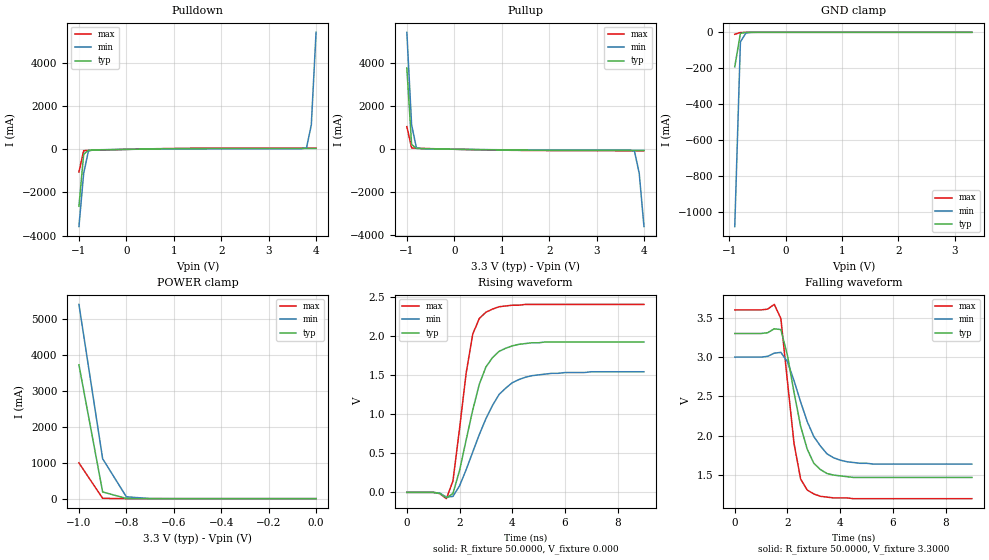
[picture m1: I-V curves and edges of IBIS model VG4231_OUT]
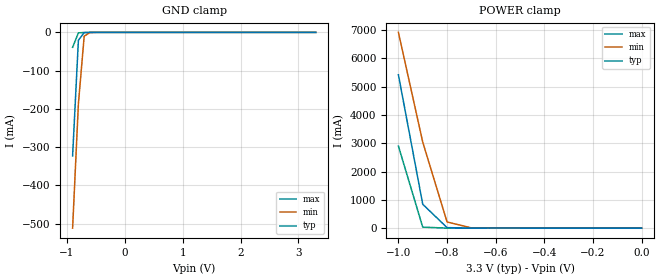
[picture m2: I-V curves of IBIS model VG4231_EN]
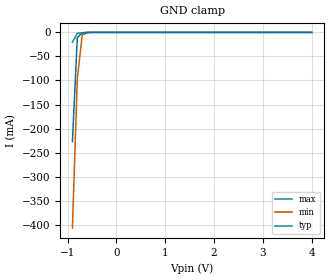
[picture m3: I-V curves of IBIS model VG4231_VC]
[IBIS ver]   2.1
[File name]   423bcacm.ibs
[File Rev]   0.1
[Date]   November 12, 2007
[Copyright]   EPSONTOYOCOM Corp.
|   Component VG-4231CAxxC
[Component]   VG-4231CAxxC
[Manufacturer]   EPSONTOYOCOM Corp.
[Package]
| variable   typ   min   max
R_pkg   0.20   0.13   0.28
L_pkg   5.16nH   4.56nH   5.76nH
C_pkg   1.23pF   1.03pF   1.53pF
[Pin]  signal_name   model_name   R_pin   L_pin   C_pin
1   VC   VG4231_VC
2   NC   NC
3   GND   GND
4   OUT   VG4231_OUT
5   OE   VG4231_EN
6   VDD   POWER
| Models and submodels in the file (3): VG4231_OUT (3-state), VG4231_EN (Input), VG4231_VC (Input)
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|   Model VG4231_OUT
[Model]   VG4231_OUT
Model_type   3-state
Polarity   Non-Inverting
Enable   Active-High
C_comp   2.2010pF   2.2010pF   2.2010pF
[Temperature Range]   27.0000   85.0000   -40.0000
[Voltage Range]   3.3000V   3.0000V   3.6000V
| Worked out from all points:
|   slope of the pulldown table from 0 to 0.495 V, typ, clamps not added: 28.4 ohm
|   slope of the pullup table from 0 to 0.495 V, typ, clamps not added: 27.7 ohm
|   GND clamp passes 1 mA (typ) near -0.71 V on its own axis
|   POWER clamp passes 1 mA (typ) near -0.71 V on its own axis
|   rising waveform, R_fixture 50.0000, V_fixture 0.000: 20-80 % time 860ps typ, 1.2ns min, 575ps max; typ from 0 V to 1.92 V
|   falling waveform, R_fixture 50.0000, V_fixture 3.3000: 20-80 % time 699ps typ, 942ps min, 507ps max; typ from 3.3 V to 1.47 V
[Pulldown]
| voltage   I(typ)   I(min)   I(max)
-1V       -2.64A     -3.58A     -1.05A
-900mV    -227mA     -1.11A     -59.8mA
-800mV    -37.8mA    -77.2mA    -45.4mA
-600mV    -24.7mA    -18.8mA    -34.3mA
1.2V      33.1mA     23.8mA     47.8mA
3.6V      41.7mA     29.9mA     59.7mA
3.8V      41.8mA     81.9mA     59.8mA
3.9V      41.9mA     1.14A      59.9mA
4V        42.4mA     5.43A      59.9mA
[Pullup]
| voltage   I(typ)   I(min)   I(max)
-1V       3.77A      5.43A      1.05A
-900mV    225mA      1.14A      61.1mA
-800mV    40.2mA     79.9mA     46.3mA
-700mV    30.8mA     27.5mA     40.2mA
-500mV    21.5mA     17.4mA     28.5mA
1.3V      -37.2mA    -28.9mA    -50.6mA
3.6V      -50.6mA    -38.5mA    -69.6mA
3.8V      -50.9mA    -91.7mA    -69.9mA
3.9V      -51.2mA    -1.12A     -70.1mA
4V        -51.8mA    -3.59A     -70.3mA
[GND_clamp]
| voltage   I(typ)   I(min)   I(max)
-900mV    -192mA     -1.08A     -11mA
-800mV    -5.99mA    -53.3mA    -1.09mA
-700mV    -646uA     -3.06mA    -314uA
3.3V      11.8pA     1.53uA     9pA
[POWER_clamp]
| voltage   I(typ)   I(min)   I(max)
-1V       3.72A      5.4A       997mA
-900mV    187mA      1.11A      9.61mA
-800mV    5.59mA     52.3mA     343uA
-700mV    457uA      3.17mA     42.4uA
-600mV    78.5uA     431uA      4.29uA
-500mV    10.7uA     85.5uA     259nA
-400mV    1.01uA     13.3uA     7.61nA
-300mV    59.2nA     1.53uA     157pA
-200mV    2.41nA     123nA      14.1pA
-100mV    84.8pA     7.1nA      11.4pA
0V        11.8pA     113pA      10.8pA
[Ramp]
| variable   typ   min   max
dV/dt_r   1.15/0.844n   0.940/1.20n   1.45/0.558n
dV/dt_f   1.10/0.697n   0.876/1.11n   1.44/0.454n
R_load = 50.0000
[Rising Waveform]
R_fixture = 50.0000
V_fixture = 0.000
V_fixture_min = 0.000
V_fixture_max = 0.000
| time   V(typ)   V(min)   V(max)
0s        204pV      8.72nV     136pV
1.5ns     -70.9mV    -60.4mV    -80.6mV
1.75ns    -14.2mV    -51.9mV    146mV
2.25ns    668mV      288mV      1.52V
2.5ns     1.05V      515mV      2.02V
2.75ns    1.38V      738mV      2.22V
3ns       1.6V       940mV      2.3V
3.5ns     1.8V       1.25V      2.37V
4.5ns     1.9V       1.47V      2.4V
9ns       1.92V      1.54V      2.4V
[Falling Waveform]
R_fixture = 50.0000
V_fixture = 3.3000
V_fixture_min = 3.0000
V_fixture_max = 3.6000
| time   V(typ)   V(min)   V(max)
0s        3.3V       3V         3.6V
1.5ns     3.36V      3.05V      3.67V
1.75ns    3.35V      3.06V      3.49V
2ns       3.02V      2.94V      2.69V
2.25ns    2.55V      2.7V       1.9V
2.5ns     2.12V      2.43V      1.45V
2.75ns    1.83V      2.18V      1.31V
3.25ns    1.57V      1.87V      1.23V
4ns       1.49V      1.69V      1.21V
9ns       1.47V      1.64V      1.2V
|   Model VG4231_EN
[Model]   VG4231_EN
Model_type   Input
Vinl =   0.6600V
Vinh =   2.6400V
C_comp   1.4070pF   1.4070pF   1.4070pF
[Temperature Range]   27.0000   85.0000   -40.0000
[Voltage Range]   3.3000V   3.0000V   3.6000V
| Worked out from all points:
|   GND clamp passes 1 mA (typ) near -0.70 V on its own axis
|   POWER clamp passes 1 mA (typ) near -0.70 V on its own axis
[GND_clamp]
| voltage   I(typ)   I(min)   I(max)
-900mV    -323mA     -512mA     -39mA
-800mV    -20.3mA    -187mA     -1.24mA
-700mV    -916uA     -9.88mA    -313uA
-600mV    -139uA     -599uA     -39.6uA
-500mV    -16.2uA    -62uA      -3.84uA
3.3V      18.4pA     290nA      -498nA
[POWER_clamp]
| voltage   I(typ)   I(min)   I(max)
-1V       5.42A      6.92A      2.9A
-900mV    844mA      3.04A      34.8mA
-800mV    18.4mA     218mA      463uA
-700mV    660uA      9.21mA     37.4uA
-600mV    72.5uA     610uA      3.68uA
-500mV    9.26uA     82.1uA     222nA
-400mV    866nA      11.7uA     6.61nA
-300mV    50.9nA     1.33uA     219pA
-200mV    2.14nA     106nA      91.4pA
-100mV    142pA      6.18nA     84.4pA
0V        74.5pA     170pA      79.2pA
|   Model VG4231_VC
[Model]   VG4231_VC
Model_type   Input
Vinl =   0.800V
Vinh =   2.000V
C_comp   1.4070pF   1.4070pF   1.4070pF
[Temperature Range]   27.0000   85.0000   -40.0000
[Voltage Range]   3.3000V   3.0000V   3.6000V
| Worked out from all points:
|   GND clamp passes 1 mA (typ) near -0.67 V on its own axis
[GND_clamp]
| voltage   I(typ)   I(min)   I(max)
-900mV    -227mA     -407mA     -20.1mA
-800mV    -11mA      -96.7mA    -2.11mA
-700mV    -1.25mA    -5.64mA    -622uA
-600mV    -265uA     -674uA     -75.4uA
-500mV    -29.8uA    -103uA     -3.49uA
4V        12.3pA     250pA      8pA
